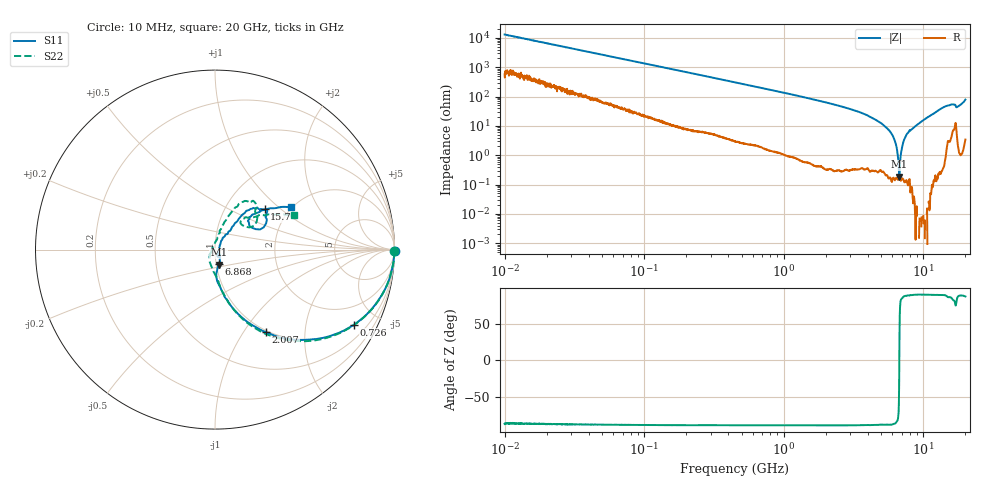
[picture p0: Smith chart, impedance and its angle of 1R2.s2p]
!Keysight Technologies,P5008B,MY61100088,A.16.20.02
!Date: Friday, August 30, 2024 10:55:14
!Correction: S11(C  2-Port  )
!S21(C  2-Port  )
!S12(C  2-Port  )
!S22(C  2-Port  )
!S2P File: Measurements: S11, S21, S12, S22:Log Frequency Sweep
# Hz S  dB  R 50
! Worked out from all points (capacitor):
!   1601 points, 10 MHz to 20 GHz, reference 50 ohm
!   read as one part in series: C = 1.22 pF near 10.39 MHz
!   lowest |Z| = 185 mohm at 6.739 GHz (marker M1)
!   series resonance near 6.725 GHz, so ESL is about 460 pH
!   S11 on the Smith chart (normalised r, x): 10 MHz: open; 726 MHz: 1.00, -3.69; 2.007 GHz: 0.98, -1.27; 6.868 GHz: 1.03, -0.16; 15.7 GHz: 1.52, +0.78; 20 GHz: 1.97, +1.22
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1e7  0.00 -0.5  -42.33 87.0  -42.32 86.9  -0.00 -0.4
3.555162e7  -0.01 -1.5  -31.46 86.7  -31.46 86.7  -0.01 -1.6
1.263918e8  -0.05 -5.4  -20.65 83.7  -20.65 83.7  -0.05 -5.5
4.472136e8  -0.47 -18.4  -10.15 70.9  -10.16 70.9  -0.47 -18.7
7.260318e8  -1.12 -28.5  -6.59 60.9  -6.59 60.9  -1.12 -28.8
1.589917e9  -3.90 -51.1  -2.31 38.2  -2.32 38.2  -3.90 -51.9
2.006635e9  -5.32 -58.3  -1.54 30.9  -1.54 30.8  -5.32 -59.4
3.465213e9  -10.05 -74.9  -0.48 14.4  -0.48 14.4  -10.02 -75.1
5.652411e9  -17.07 -87.3  -0.09 0.3  -0.09 0.2  -17.21 -90.1
6.738606e9  -21.21 -75.8  -0.02 -4.7  -0.02 -4.8  -21.71 -108.7
6.867879e9  -21.81 -73.6  -0.02 -5.2  -0.02 -5.4  -22.32 -112.0
7.844959e9  -26.48 -56.2  0.01 -9.1  0.01 -9.2  -27.49 -133.4
9.577292e9  -32.69 -12.9  0.03 -15.5  0.03 -15.6  -34.95 160.3
9.948277e9  -31.42 25.2  0.03 -16.8  0.03 -17.0  -33.22 112.0
1.104427e10  -22.73 55.0  0.02 -20.9  0.01 -21.0  -23.11 77.5
1.273595e10  -14.33 52.2  -0.12 -27.3  -0.12 -27.5  -14.40 68.8
1.407205e10  -10.40 48.8  -0.34 -32.9  -0.33 -33.1  -10.55 61.1
1.569675e10  -8.98 39.1  -0.78 -38.3  -0.78 -38.6  -9.30 52.4
1.638242e10  -9.24 33.8  -1.04 -38.8  -1.04 -39.1  -9.89 44.8
1.767617e10  -12.29 41.0  -0.39 -40.1  -0.39 -40.3  -12.79 47.6
1.871311e10  -10.28 41.5  -0.48 -47.8  -0.48 -48.1  -10.36 38.2
2e10  -6.29 29.2  -1.39 -59.7  -1.38 -60.0  -6.40 23.7
